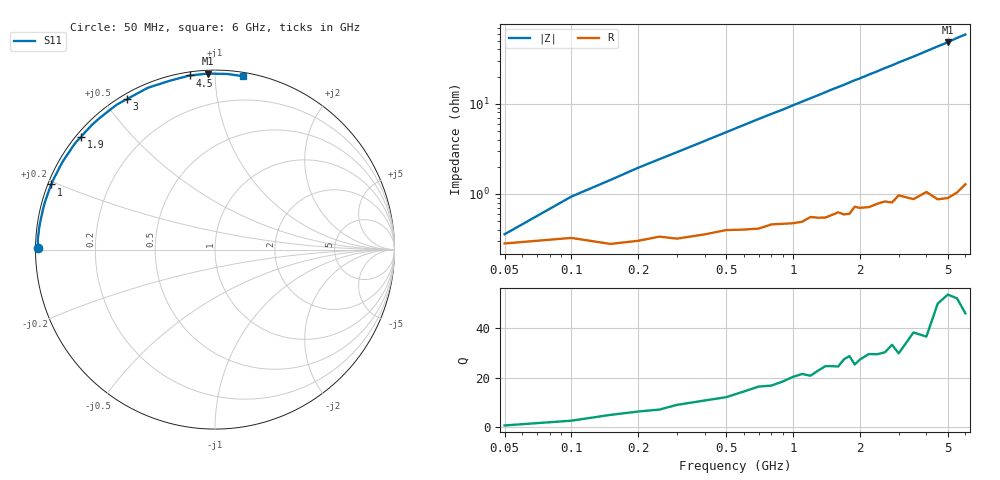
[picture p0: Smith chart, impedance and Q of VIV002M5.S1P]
! Infineon Technologies  Discrete & RF Semiconductors
! BB 804
! Si Tuning Diode in SOT23
! VR =
! S-Parameters:  July  1999
# GHz  S  MA  R  50
!  f  S11
! GHz  MAG  ANG
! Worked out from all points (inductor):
!   34 points, 50 MHz to 6 GHz, reference 50 ohm
!   read as one part to ground: L = 1.53 nH near 150 MHz
!   highest Q = 51.9 at 5 GHz (marker M1), where L = 1.53 nH
!   S11 on the Smith chart (normalised r, x): 50 MHz: 0.01, +0.00; 1 GHz: 0.01, +0.19; 1.9 GHz: 0.01, +0.36; 3 GHz: 0.02, +0.57; 4.5 GHz: 0.02, +0.86; 6 GHz: 0.03, +1.17
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0.05  0.9888 179.5
0.1  0.9871 178.0
0.15  0.9889 176.8
0.2  0.988 175.6
0.4  0.986 171.2
0.6  0.9843 166.8
0.8  0.9823 162.5
0.9  0.9821 160.5
1  0.982 158.3
1.1  0.9814 156.2
1.4  0.9799 150.0
1.5  0.9787 147.9
1.6  0.9774 146.0
1.7  0.9788 144.1
1.8  0.9788 142.0
1.9  0.9749 140.0
2  0.9759 138.3
2.2  0.9761 134.4
2.4  0.9746 130.9
2.6  0.9739 127.1
2.8  0.9753 123.9
3  0.9714 120.3
3.5  0.9761 112.6
4  0.9739 105.1
4.5  0.9803 98.3
5  0.9815 92.3
5.5  0.981 85.9
6  0.9787 80.9
